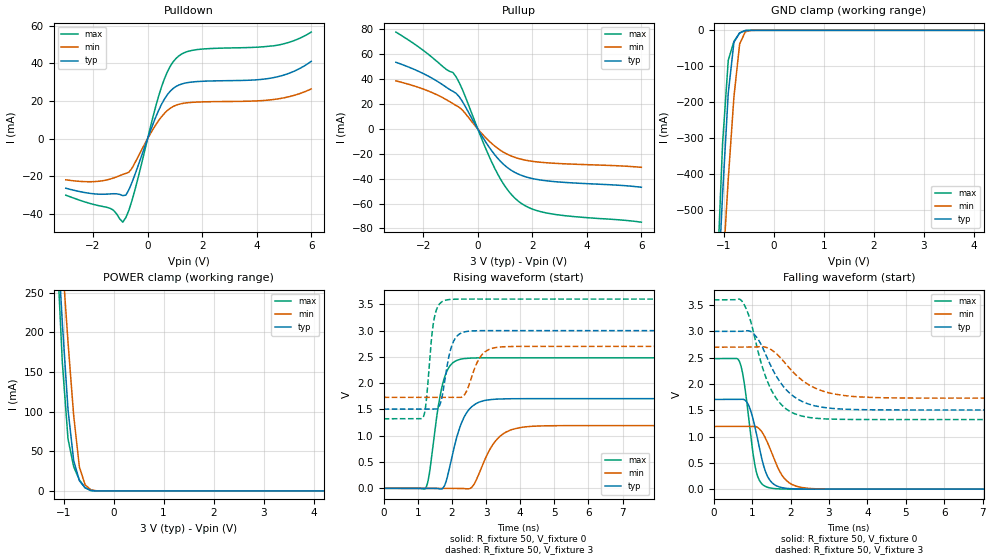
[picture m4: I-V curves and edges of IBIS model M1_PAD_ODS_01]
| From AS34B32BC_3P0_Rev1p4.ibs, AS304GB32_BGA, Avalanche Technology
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[Model] M1_PAD_ODS_01
Model_type I/O
Enable   Active-High
Vinl  =  0.8
Vinh  =  2.2
Vmeas =  1.5
Cref  =  30e-12
| Capacitance  typ   min   max
C_comp   6.128805e-12   5.681079e-12   6.591827e-12
| Variables   typ   min   max
[GND Clamp Reference]   0   0   0
[POWER Clamp Reference]   3   2.7   3.6
[Pulldown Reference]   0   0   0
[Pullup Reference]   3   2.7   3.6
[Temperature Range]   25   125   -40
[Voltage Range]   3   2.7   3.6
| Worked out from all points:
|   slope of the pulldown table from 0 to 0.45 V, typ, clamps not added: 27.4 ohm
|   slope of the pullup table from 0 to 0.45 V, typ, clamps not added: 28.8 ohm
|   GND clamp passes 1 mA (typ) near -0.57 V on its own axis
|   POWER clamp passes 1 mA (typ) near -0.47 V on its own axis
|   falling waveform, R_fixture 50, V_fixture 0: 20-80 % time 331ps typ, 446ps min, 260ps max; typ from 1.71 V to 0 V
|   falling waveform, R_fixture 50, V_fixture 3: 20-80 % time 744ps typ, 902ps min, 602ps max; typ from 3 V to 1.51 V
|   rising waveform, R_fixture 50, V_fixture 0: 20-80 % time 454ps typ, 583ps min, 344ps max; typ from 0 V to 1.71 V
|   rising waveform, R_fixture 50, V_fixture 3: 20-80 % time 261ps typ, 361ps min, 192ps max; typ from 1.51 V to 3 V
[GND Clamp]
| Voltage   I(typ)   I(min)   I(max)
-3V       -6.848A    -5.961A    -8.2A
-1.138V   -783.9mA   -953.3mA   -701.6mA
-1.024V   -456.3mA   -675.8mA   -315.2mA
-910.3mV  -174.6mA   -413.8mA   -83.06mA
-796.6mV  -33.06mA   -184.3mA   -30.65mA
-682.8mV  -7.332mA   -38.2mA    -7.06mA
-569mV    -713uA     -3.879mA   -286.8uA
-455.2mV  -15.31uA   -289.9uA   -1.608uA
6V        0A         0A         0A
[POWER Clamp]
| Voltage   I(typ)   I(min)   I(max)
-3V       2.695A     2.364A     3.234A
-1.138V   339.1mA    399.9mA    313.8mA
-1.024V   212.3mA    291.5mA    162.2mA
-910.3mV  102.5mA    187.9mA    65.61mA
-796.6mV  38.13mA    95.01mA    30.53mA
-682.8mV  12.94mA    30.26mA    13.87mA
-569mV    3.981mA    7.764mA    4.118mA
-455.2mV  618.9uA    1.561mA    450.1uA
-227.6mV  142.3nA    9.251uA    10.37nA
6V        0A         0A         0A
[Pulldown]
| Voltage   I(typ)   I(min)   I(max)
-3V       -26.36mA   -21.88mA   -30.04mA
-1.366V   -29.37mA   -21.44mA   -37.07mA
-910.3mV  -30.26mA   -19.02mA   -44.4mA
-796.6mV  -30.03mA   -18.45mA   -41.9mA
-569mV    -23.1mA    -15.63mA   -32.68mA
206.9mV   8.128mA    5.203mA    12.16mA
517.2mV   18.44mA    11.77mA    27.81mA
724.1mV   23.38mA    14.96mA    35.49mA
1.034V    27.67mA    17.73mA    42.54mA
1.759V    30.28mA    19.41mA    47.23mA
4.614V    32.42mA    20.8mA     49.33mA
6V        41.08mA    26.43mA    56.64mA
[Pullup]
| Voltage   I(typ)   I(min)   I(max)
-3V       53.53mA    38.58mA    77.79mA
-1.821V   42.49mA    30.53mA    60.12mA
-910.3mV  30.2mA     20.33mA    45.32mA
-796.6mV  28.64mA    18.81mA    41.96mA
-569mV    22.26mA    15.27mA    32mA
206.9mV   -7.586mA   -5.1mA     -11.3mA
620.7mV   -20.68mA   -13.72mA   -31.55mA
1.034V    -30.14mA   -19.8mA    -47.15mA
1.552V    -36.89mA   -24.12mA   -59.12mA
2.069V    -40.18mA   -26.23mA   -64.93mA
2.69V     -42.09mA   -27.45mA   -68.2mA
6V        -46.88mA   -30.86mA   -74.95mA
[Ramp]
dV/dt_r   1.02353/0.453554n  0.715782/0.582767n  1.4895/0.344067n
dV/dt_f   0.896545/0.744408n  0.581576/0.901957n  1.3662/0.60195n
R_load = 50
[Falling Waveform]
R_fixture = 50
V_fixture = 0
V_fixture_min = 0
V_fixture_max = 0
| Time   V(typ)   V(min)   V(max)
0s        1.706V     1.193V     2.482V
665.2ps   1.707V     1.194V     2.433V
770.5ps   1.708V     1.194V     2.126V
893.8ps   1.616V     1.194V     1.455V
1.104ns   1.078V     1.188V     339.8mV
1.334ns   360.4mV    987.3mV    55.8mV
1.531ns   114.2mV    651.1mV    14.73mV
1.909ns   14.73mV    152.1mV    1.649mV
2.629ns   693uV      8.132mV    831.5uV
21.88ns   19.91nV    439.8nV    13.87nV
[Falling Waveform]
R_fixture = 50
V_fixture = 3
V_fixture_min = 2.7
V_fixture_max = 3.6
| Time   V(typ)   V(min)   V(max)
0s        3V         2.7V       3.6V
737.6ps   3.002V     2.701V     3.572V
913ps     3.01V      2.701V     3.305V
1.115ns   2.891V     2.706V     2.733V
1.511ns   2.308V     2.646V     1.869V
1.928ns   1.859V     2.337V     1.504V
2.455ns   1.622V     1.994V     1.366V
3.313ns   1.524V     1.788V     1.328V
4.577ns   1.507V     1.736V     1.324V
21.88ns   1.506V     1.731V     1.323V
[Rising Waveform]
R_fixture = 50
V_fixture = 0
V_fixture_min = 0
V_fixture_max = 0
| Time   V(typ)   V(min)   V(max)
0s        15.01nV    251.3nV    41.19nV
1.229ns   -269.3uV   -346.3uV   3.046mV
1.337ns   -293uV     -376.8uV   265.4mV
1.574ns   -3.494mV   -443.6uV   1.446V
1.769ns   34.4mV     -498.8uV   2.08V
2.336ns   1.325V     -4.578mV   2.466V
2.622ns   1.572V     49.83mV    2.479V
3.364ns   1.698V     962.3mV    2.482V
4.141ns   1.705V     1.168V     2.482V
21.88ns   1.706V     1.193V     2.482V
[Rising Waveform]
R_fixture = 50
V_fixture = 3
V_fixture_min = 2.7
V_fixture_max = 3.6
| Time   V(typ)   V(min)   V(max)
0s        1.506V     1.731V     1.323V
1.158ns   1.507V     1.731V     1.351V
1.241ns   1.507V     1.731V     1.613V
1.493ns   1.506V     1.731V     3.267V
1.677ns   1.646V     1.731V     3.535V
1.86ns    2.328V     1.732V     3.586V
2.224ns   2.937V     1.731V     3.599V
2.892ns   2.999V     2.549V     3.6V
3.499ns   2.999V     2.692V     3.6V
21.88ns   3V         2.7V       3.6V
